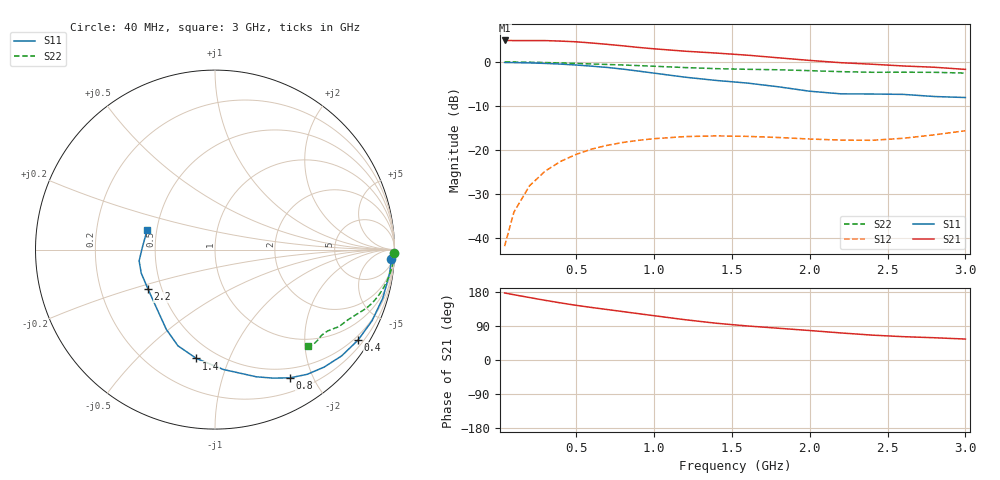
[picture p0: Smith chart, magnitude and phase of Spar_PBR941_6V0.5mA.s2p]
! Filename:  PBR941J.S2P  Version:  3.0
! NXP part #:  PBR941  Date: July 1998
! Bias condition:  Vce=6V, Ic=0.5mA
#  MHz  S  MA  R 50
! Freq  S11  S21  S12  S22
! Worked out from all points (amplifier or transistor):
!   21 points, 40 MHz to 3 GHz, reference 50 ohm
!   highest |S21| = 4.9 dB at 40 MHz (marker M1)
!   |S21| within 3 dB of that: start of sweep to 1.456 GHz
!   unconditionally stable (mu >= 1): 2.036 GHz to end of sweep
!   at 300 MHz: K = 0.13, MSG = 14.8 dB, |S12| = -24.8 dB
!   at 1 GHz: K = 0.41, MSG = 10.2 dB, |S12| = -17.4 dB
!   at 3 GHz: K = 1.17, MAG = 4.5 dB, |S12| = -15.6 dB
!   lowest NFmin = 0.94 dB at 900 MHz
!   S11 on the Smith chart (normalised r, x): 40 MHz: 9, -34; 400 MHz: 0.37, -3.42; 800 MHz: 0.37, -1.68; 1.4 GHz: 0.39, -0.76; 2.2 GHz: 0.42, -0.23; 3 GHz: 0.44, +0.12
40  0.9846 -3.2  1.751 176.9  0.008062 88.4  0.999 -1.2
100  0.9813 -8.0  1.746 172.3  0.01969 86.0  0.9969 -2.8
200  0.9734 -16.1  1.747 164.8  0.03908 79.6  0.9909 -5.6
300  0.9607 -24.3  1.745 157.5  0.05734 75.6  0.9824 -8.4
400  0.9432 -32.3  1.722 150.7  0.07414 71.2  0.9715 -11.0
500  0.9211 -40.0  1.69 144.2  0.08896 67.4  0.9597 -13.4
600  0.8934 -47.1  1.638 138.6  0.1022 63.6  0.9471 -15.5
700  0.8641 -53.5  1.582 133.1  0.1128 60.5  0.9344 -17.5
800  0.8274 -59.8  1.521 127.7  0.1215 57.3  0.9215 -19.2
900  0.7854 -65.7  1.459 122.3  0.1285 54.8  0.9073 -20.8
1000  0.7452 -72.0  1.407 116.9  0.1341 52.1  0.892 -22.3
1200  0.6697 -86.0  1.322 106.3  0.1417 47.6  0.8618 -25.1
1400  0.6151 -99.8  1.259 97.0  0.1443 44.2  0.8375 -27.9
1600  0.5743 -111.1  1.191 89.8  0.1425 43.4  0.8234 -30.1
1800  0.5207 -121.4  1.112 83.8  0.1383 45.1  0.8133 -31.9
2000  0.4641 -133.8  1.039 77.8  0.1329 47.5  0.7952 -33.6
2200  0.4333 -149.3  0.9788 71.4  0.1293 51.7  0.7742 -35.8
2400  0.4315 -162.3  0.9404 65.7  0.1285 58.1  0.7618 -38.8
2600  0.4273 -171.6  0.8985 61.6  0.1355 66.2  0.7628 -41.7
2800  0.4042 177.8  0.8689 58.7  0.1483 73.6  0.7611 -43.9
3000  0.3934 163.5  0.8213 55.3  0.1651 79.2  0.7455 -45.9
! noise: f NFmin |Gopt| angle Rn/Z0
500  1.376  0.696  23.53  0.848
900  0.935  0.716  30.55  0.695
1000  1.377  0.661  41.13  0.68
2000  2.475  0.497  108  0.344
